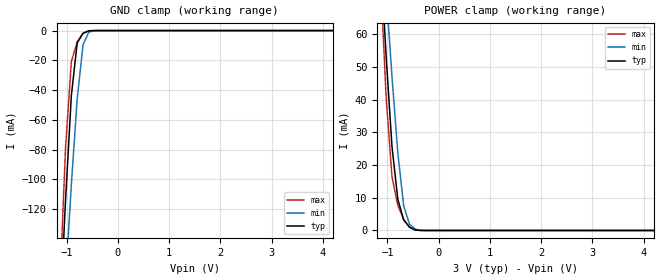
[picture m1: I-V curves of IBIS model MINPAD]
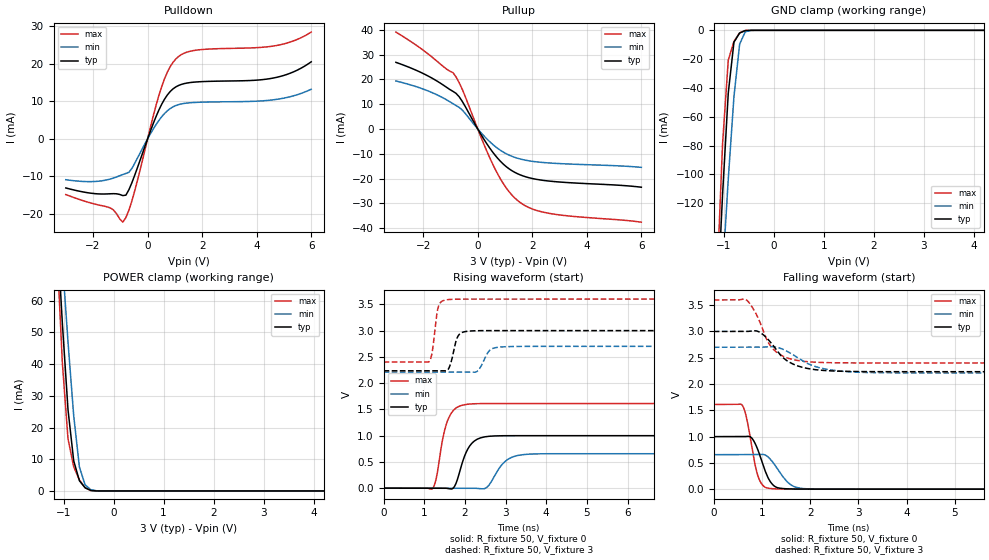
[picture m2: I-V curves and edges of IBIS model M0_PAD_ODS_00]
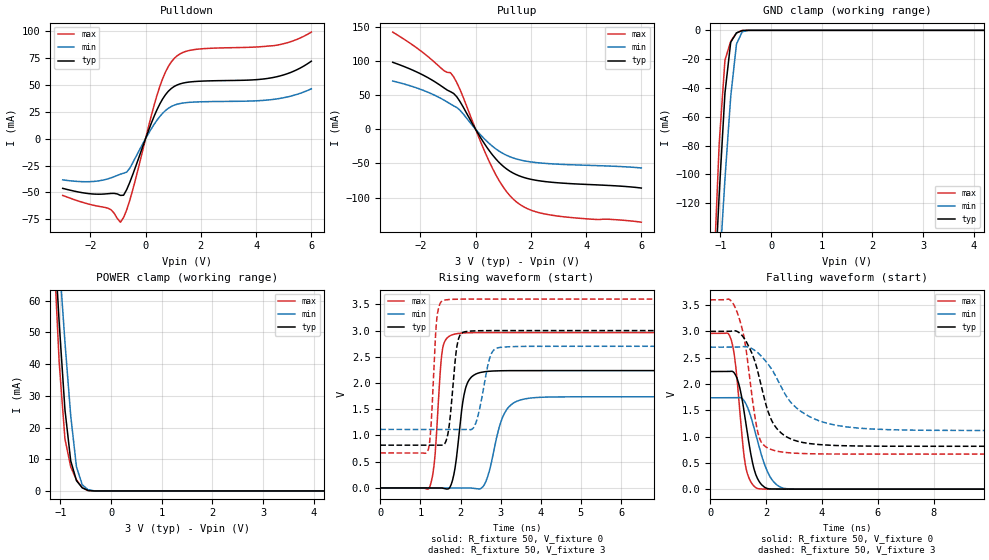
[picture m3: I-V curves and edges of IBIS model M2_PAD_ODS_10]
| Created by SiliconSmart  O-2018.09-SP2-3
[IBIS Ver]   4.0
[File Name]   as31b32bc_3p0_rev1p4.ibs
[File Rev]   1.4
[Date]   Thursday Mar 21 2024
|[Source]   Avalanche Team
|[Notes]   Generated IBIS models from Silicon Smart
|[Rev 1.0]  Initial Release based on extracted netlist
|   Characterization
|[Rev 1.1]  Recharacterization with Hspice, run in high accuracy mode
|[Rev 1.2]  Recharacterization with Hspice, run with parameters inline
|   with the datasheet
|[Rev 1.3]  Recharacterization with Hspice, run with updated VIH/VIL
|   in parallel with datasheet rev X.7
|[Rev 1.4]  Update the pin to the package pinout assignment
|[Disclaimer]   THE MODEL LIBRARIES ARE PROVIDED AS IS.
|[Copyright]   Copyright 2019, Avalanche Technology., All Rights Reserved
[Component]   AS301GB32_BGA
[Manufacturer] Avalanche Technology
| CONTENT :
| This file contains IBIS MODEL for PSRAM device
| AS301GB32
| USAGE :
| The models are derived for the 2.7V to 3.6V I/O Operation.
| Temperatures for model generation: typ: 25, max: -40, min: 125
| Voltages : typ: 3.0V, min: 2.7V, max: 3.6V
| PACKAGES SUPPORTED :
| 142-ball FBGA (15mm x 17mm)
| VERIFICATION
| Errors  : 0
| Warnings: 16
| All warnings due to non-monotonic data:
[Package]
R_pkg  0   0   0
L_pkg  0   0   0
C_pkg  0   0   0
[Pin]   signal_name   model_name   R_pin   L_pin   C_pin
P8   E#   MINPAD   0.254	7.307E-9	1.178E-12
P7   G#   MINPAD   0.243	7.052E-9	1.094E-12
J2   CR#   MINPAD   0.547	10.386E-9	1.789E-12
K3   PG#   MINPAD   0.451	10.329E-9	1.676E-12
M8   W#   MINPAD   0.377	9.020E-9	1.417E-12
M2   ADDR_26   MINPAD   0.425	9.037E-9	1.604E-12
L4   ADDR_25   MINPAD   0.419	9.644E-9	1.527E-12
K13   ADDR_24   MINPAD   0.495	9.978E-9	1.745E-12
M3   ADDR_23   MINPAD   0.371	9.313E-9	1.466E-12
L3   ADDR_22   MINPAD   0.412	9.753E-9	1.540E-12
M7   ADDR_21   MINPAD   0.368	8.765E-9	1.384E-12
P12   ADDR_20   MINPAD   0.287	8.287E-9	1.639E-12
L12   ADDR_19   MINPAD   0.424	10.320E-9	1.620E-12
N11   ADDR_18   MINPAD   0.338	8.691E-9	1.470E-12
N6   ADDR_17   MINPAD   0.309	8.196E-9	1.279E-12
P6   ADDR_16   MINPAD   0.256	7.462E-9	1.204E-12
L13   ADDR_15   MINPAD   0.463	10.719E-9	1.740E-12
M13   ADDR_14   MINPAD   0.421	10.290E-9	1.689E-12
P10   ADDR_13   MINPAD   0.262	7.671E-9	1.349E-12
N10   ADDR_12   MINPAD   0.340	8.540E-9	1.360E-12
M12   ADDR_11   MINPAD   0.402	9.876E-9	1.604E-12
N13   ADDR_10   MINPAD   0.399	9.819E-9	1.696E-12
L11   ADDR_9   MINPAD   0.443	9.732E-9	1.569E-12
M11   ADDR_8   MINPAD   0.436	9.682E-9	1.671E-12
P5   ADDR_7   MINPAD   0.253	7.464E-9	1.277E-12
P3   ADDR_6   MINPAD   0.279	8.031E-9	1.557E-12
N5   ADDR_5   MINPAD   0.313	8.320E-9	1.359E-12
N4   ADDR_4   MINPAD   0.329	8.138E-9	1.428E-12
M4   ADDR_3   MINPAD   0.379	8.543E-9	1.406E-12
N2   ADDR_2   MINPAD   0.378	9.572E-9	1.637E-12
N9   ADDR_1   MINPAD   0.315	8.416E-9	1.305E-12
M9   ADDR_0   MINPAD   0.403	9.225E-9	1.473E-12
E2   DQ_31   MIOPAD   0.365	8.798E-9	1.454E-12
F2   DQ_30   MIOPAD   0.418	9.057E-9	1.576E-12
D2   DQ_29   MIOPAD   0.358	8.697E-9	1.520E-12
E3   DQ_28   MIOPAD   0.348	8.812E-9	1.441E-12
E12   DQ_27   MIOPAD   0.327	8.506E-9	1.443E-12
D10   DQ_26   MIOPAD   0.309	7.715E-9	1.264E-12
C9   DQ_25   MIOPAD   0.279	7.395E-9	1.219E-12
C7   DQ_24   MIOPAD   0.252	6.802E-9	1.108E-12
G4   DQ_23   MIOPAD   0.455	10.071E-9	1.775E-12
G3   DQ_22   MIOPAD   0.457	10.100E-9	1.750E-12
F13   DQ_21   MIOPAD   0.377	9.387E-9	1.566E-12
D13   DQ_20   MIOPAD   0.295	8.231E-9	1.460E-12
C10   DQ_19   MIOPAD   0.293	7.553E-9	1.298E-12
E8   DQ_18   MIOPAD   0.393	8.323E-9	1.436E-12
F6   DQ_17   MIOPAD   0.425	8.913E-9	1.517E-12
E5   DQ_16   MIOPAD   0.379	8.982E-9	1.460E-12
E13   DQ_15   MIOPAD   0.363	8.555E-9	1.474E-12
G11   DQ_14   MIOPAD   0.475	9.536E-9	1.630E-12
E10   DQ_13   MIOPAD   0.404	8.563E-9	1.453E-12
F9   DQ_12   MIOPAD   0.409	9.347E-9	1.513E-12
C8   DQ_11   MIOPAD   0.257	6.782E-9	1.111E-12
C6   DQ_10   MIOPAD   0.238	7.000E-9	1.114E-12
D6   DQ_9   MIOPAD   0.292	7.776E-9	1.248E-12
D4   DQ_8   MIOPAD   0.305	7.782E-9	1.343E-12
G12   DQ_7   MIOPAD   0.502	10.055E-9	1.687E-12
C12   DQ_6   MIOPAD   0.275	7.857E-9	1.346E-12
D11   DQ_5   MIOPAD   0.286	7.835E-9	1.360E-12
D9   DQ_4   MIOPAD   0.306	8.035E-9	1.299E-12
E7   DQ_3   MIOPAD   0.384	8.178E-9	1.375E-12
C5   DQ_2   MIOPAD   0.231	6.786E-9	1.150E-12
D5   DQ_1   MIOPAD   0.307	7.698E-9	1.346E-12
C3   DQ_0   MIOPAD   0.267	7.420E-9	1.241E-12
G13   INT#   MIOPAD   0.480	10.704E-9	1.759E-12
F10   VSSIO   GND   NA   NA   NA
L10   VSSIO   GND   NA   NA   NA
E9   VSSIO   GND   NA   NA   NA
L9   VSSIO   GND   NA   NA   NA
F8   VSSIO   GND   NA   NA   NA
L8   VSSIO   GND   NA   NA   NA
F7   VSSIO   GND   NA   NA   NA
L7   VSSIO   GND   NA   NA   NA
E6   VSSIO   GND   NA   NA   NA
L6   VSSIO   GND   NA   NA   NA
G5   VSSIO   GND   NA   NA   NA
A14   VSS   GND   NA   NA   NA
B14   VSS   GND   NA   NA   NA
C14   VSS   GND   NA   NA   NA
H13   VSS   GND   NA   NA   NA
R14   VSS   GND   NA   NA   NA
T14   VSS   GND   NA   NA   NA
A13   VSS   GND   NA   NA   NA
T13   VSS   GND   NA   NA   NA
A12   VSS   GND   NA   NA   NA
G10   VSS   GND   NA   NA   NA
H10   VSS   GND   NA   NA   NA
J10   VSS   GND   NA   NA   NA
K10   VSS   GND   NA   NA   NA
F5   VSS   GND   NA   NA   NA
L5   VSS   GND   NA   NA   NA
A2   VSS   GND   NA   NA   NA
T2   VSS   GND   NA   NA   NA
A1   VSS   GND   NA   NA   NA
B1   VSS   GND   NA   NA   NA
R1   VSS   GND   NA   NA   NA
T1   VSS   GND   NA   NA   NA
F12   VCCIO   POWER   NA   NA   NA
J12   VCCIO   POWER   NA   NA   NA
E11   VCCIO   POWER   NA   NA   NA
M10   VCCIO   POWER   NA   NA   NA
D8   VCCIO   POWER   NA   NA   NA
N8   VCCIO   POWER   NA   NA   NA
D7   VCCIO   POWER   NA   NA   NA
N7   VCCIO   POWER   NA   NA   NA
M5   VCCIO   POWER   NA   NA   NA
E4   VCCIO   POWER   NA   NA   NA
F3   VCCIO   POWER   NA   NA   NA
J3   VCCIO   POWER   NA   NA   NA
C13   VCC   POWER   NA   NA   NA
P13   VCC   POWER   NA   NA   NA
D12   VCC   POWER   NA   NA   NA
N12   VCC   POWER   NA   NA   NA
C11   VCC   POWER   NA   NA   NA
F11   VCC   POWER   NA   NA   NA
H11   VCC   POWER   NA   NA   NA
J11   VCC   POWER   NA   NA   NA
K11   VCC   POWER   NA   NA   NA
P11   VCC   POWER   NA   NA   NA
C4   VCC   POWER   NA   NA   NA
F4   VCC   POWER   NA   NA   NA
H4   VCC   POWER   NA   NA   NA
J4   VCC   POWER   NA   NA   NA
K4   VCC   POWER   NA   NA   NA
P4   VCC   POWER   NA   NA   NA
D3   VCC   POWER   NA   NA   NA
N3   VCC   POWER   NA   NA   NA
C2   VCC   POWER   NA   NA   NA
P2   VCC   POWER   NA   NA   NA
| IOPAD
[Model Selector] MIOPAD
| Model Description
M0_PAD_ODS_00   ODS_00
M1_PAD_ODS_01   ODS_01
M2_PAD_ODS_10   ODS_10
M3_PAD_ODS_11   ODS_11
| Models and submodels in the file (5): MINPAD (Input), M0_PAD_ODS_00 (I/O), M2_PAD_ODS_10 (I/O), M1_PAD_ODS_01 (I/O), M3_PAD_ODS_11 (I/O)
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[Model] MINPAD
Model_type Input
Enable   Active-High
Vinl  =  0.8
Vinh  =  2.2
| Capacitance  typ   min   max
C_comp   1.532639e-12   1.418869e-12   1.647023e-12
| Variables   typ   min   max
[GND Clamp Reference]   0   0   0
[POWER Clamp Reference]   3   2.7   3.6
[Pulldown Reference]   0   0   0
[Pullup Reference]   3   2.7   3.6
[Temperature Range]   25   125   -40
[Voltage Range]   3   2.7   3.6
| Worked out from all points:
|   GND clamp passes 1 mA (typ) near -0.63 V on its own axis
|   POWER clamp passes 1 mA (typ) near -0.57 V on its own axis
[GND Clamp]
| Voltage   I(typ)   I(min)   I(max)
-3V       -1.712A    -1.49A     -2.05A
-1.138V   -196mA     -238.3mA   -175.4mA
-1.024V   -114.1mA   -169mA     -78.79mA
-910.3mV  -43.65mA   -103.4mA   -20.76mA
-796.6mV  -8.265mA   -46.07mA   -7.662mA
-682.8mV  -1.833mA   -9.55mA    -1.764mA
-569mV    -178.2uA   -969.7uA   -71.6uA
-455.2mV  -3.827uA   -72.47uA   -401.3nA
6V        0A         0A         0A
[POWER Clamp]
| Voltage   I(typ)   I(min)   I(max)
-3V       673.8mA    591mA      808.5mA
-1.138V   84.79mA    99.96mA    78.44mA
-1.024V   53.08mA    72.89mA    40.56mA
-910.3mV  25.62mA    46.98mA    16.4mA
-796.6mV  9.531mA    23.75mA    7.632mA
-682.8mV  3.235mA    7.564mA    3.468mA
-569mV    995.3uA    1.941mA    1.029mA
-455.2mV  154.7uA    390.4uA    112.5uA
-227.6mV  35.58nA    2.313uA    2.593nA
6V        0A         0A         0A
[Model] M0_PAD_ODS_00
Model_type I/O
Enable   Active-High
Vinl  =  0.8
Vinh  =  2.2
Vmeas =  1.5
Cref  =  30e-12
| Capacitance  typ   min   max
C_comp   1.536816e-12   1.424706e-12   1.652746e-12
| Variables   typ   min   max
[GND Clamp Reference]   0   0   0
[POWER Clamp Reference]   3   2.7   3.6
[Pulldown Reference]   0   0   0
[Pullup Reference]   3   2.7   3.6
[Temperature Range]   25   125   -40
[Voltage Range]   3   2.7   3.6
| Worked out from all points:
|   slope of the pulldown table from 0 to 0.45 V, typ, clamps not added: 54.7 ohm
|   slope of the pullup table from 0 to 0.45 V, typ, clamps not added: 57.3 ohm
|   GND clamp passes 1 mA (typ) near -0.63 V on its own axis
|   POWER clamp passes 1 mA (typ) near -0.57 V on its own axis
|   falling waveform, R_fixture 50, V_fixture 0: 20-80 % time 244ps typ, 320ps min, 198ps max; typ from 1 V to 0 V
|   falling waveform, R_fixture 50, V_fixture 3: 20-80 % time 499ps typ, 644ps min, 396ps max; typ from 3 V to 2.23 V
|   rising waveform, R_fixture 50, V_fixture 0: 20-80 % time 285ps typ, 362ps min, 248ps max; typ from 0 V to 1 V
|   rising waveform, R_fixture 50, V_fixture 3: 20-80 % time 146ps typ, 198ps min, 114ps max; typ from 2.23 V to 3 V
[GND Clamp]
| Voltage   I(typ)   I(min)   I(max)
-3V       -1.712A    -1.49A     -2.05A
-1.138V   -196mA     -238.3mA   -175.4mA
-1.024V   -114.1mA   -169mA     -78.8mA
-910.3mV  -43.65mA   -103.4mA   -20.77mA
-796.6mV  -8.267mA   -46.07mA   -7.668mA
-682.8mV  -1.833mA   -9.55mA    -1.767mA
-569mV    -178.4uA   -969.7uA   -71.94uA
-455.2mV  -3.831uA   -72.48uA   -403.8nA
6V        0A         0A         0A
[POWER Clamp]
| Voltage   I(typ)   I(min)   I(max)
-3V       673.8mA    591mA      808.5mA
-1.138V   84.79mA    99.96mA    78.44mA
-1.024V   53.08mA    72.89mA    40.56mA
-910.3mV  25.62mA    46.98mA    16.4mA
-796.6mV  9.531mA    23.75mA    7.632mA
-682.8mV  3.235mA    7.564mA    3.468mA
-569mV    995.3uA    1.941mA    1.029mA
-455.2mV  154.7uA    390.4uA    112.5uA
-227.6mV  35.58nA    2.313uA    2.593nA
6V        0A         0A         0A
[Pulldown]
| Voltage   I(typ)   I(min)   I(max)
-3V       -13.11mA   -10.91mA   -14.87mA
-1.366V   -14.66mA   -10.71mA   -18.44mA
-910.3mV  -15.13mA   -9.525mA   -22.23mA
-796.6mV  -15.02mA   -9.239mA   -20.99mA
-569mV    -11.56mA   -7.817mA   -16.37mA
206.9mV   4.069mA    2.602mA    6.097mA
517.2mV   9.226mA    5.888mA    13.93mA
724.1mV   11.7mA     7.479mA    17.77mA
1.034V    13.84mA    8.867mA    21.28mA
1.759V    15.14mA    9.703mA    23.62mA
4.614V    16.21mA    10.4mA     24.74mA
6V        20.54mA    13.21mA    28.45mA
[Pullup]
| Voltage   I(typ)   I(min)   I(max)
-3V       26.89mA    19.37mA    39.1mA
-1.821V   21.37mA    15.34mA    30.28mA
-910.3mV  15.2mA     10.23mA    22.74mA
-796.6mV  14.37mA    9.461mA    21.03mA
-569mV    11.16mA    7.659mA    16.04mA
206.9mV   -3.805mA   -2.558mA   -5.667mA
620.7mV   -10.37mA   -6.883mA   -15.82mA
1.034V    -15.12mA   -9.936mA   -23.64mA
1.552V    -18.5mA    -12.1mA    -29.65mA
2.069V    -20.15mA   -13.16mA   -32.55mA
2.69V     -21.11mA   -13.77mA   -34.19mA
6V        -23.51mA   -15.49mA   -37.63mA
[Ramp]
dV/dt_r   0.59988/0.284835n  0.393696/0.362182n  0.967082/0.24767n
dV/dt_f   0.45937/0.498633n  0.294233/0.644316n  0.719379/0.396117n
R_load = 50
[Falling Waveform]
R_fixture = 50
V_fixture = 0
V_fixture_min = 0
V_fixture_max = 0
| Time   V(typ)   V(min)   V(max)
0s        999.8mV    656.2mV    1.612V
592.6ps   1V         656.6mV    1.594V
662.7ps   1.002V     656.6mV    1.423V
775ps     985mV      656.7mV    887.5mV
920.8ps   732.5mV    658.3mV    236.4mV
1.05ns    387.5mV    655.1mV    44.33mV
1.221ns   87.43mV    516.2mV    8.708mV
1.592ns   4.378mV    87.01mV    1.102mV
2.018ns   780.3uV    4.7mV      706uV
21.88ns   13.06nV    -2.279uV   3.818uV
[Falling Waveform]
R_fixture = 50
V_fixture = 3
V_fixture_min = 2.7
V_fixture_max = 3.6
| Time   V(typ)   V(min)   V(max)
0s        3V         2.7V       3.6V
662.6ps   3.001V     2.701V     3.609V
930.9ps   2.997V     2.701V     3.233V
1.117ns   2.859V     2.709V     2.815V
1.233ns   2.732V     2.709V     2.664V
1.556ns   2.422V     2.604V     2.487V
2.006ns   2.286V     2.366V     2.42V
2.5ns     2.247V     2.259V     2.405V
3.502ns   2.235V     2.214V     2.401V
21.88ns   2.234V     2.21V      2.401V
[Rising Waveform]
R_fixture = 50
V_fixture = 0
V_fixture_min = 0
V_fixture_max = 0
| Time   V(typ)   V(min)   V(max)
0s        6.54nV     88.47nV    -73.19nV
1.207ns   -456.9uV   -520.5uV   -4.427mV
1.285ns   -486.5uV   -554.2uV   157.9mV
1.593ns   -8.932mV   -686.9uV   1.324V
1.775ns   80.53mV    -765.4uV   1.522V
2.069ns   743.7mV    -892.4uV   1.599V
2.519ns   980.4mV    5.17mV     1.611V
2.991ns   998.7mV    510.2mV    1.611V
3.605ns   998.9mV    648.6mV    1.611V
21.88ns   999.8mV    656.2mV    1.612V
[Rising Waveform]
R_fixture = 50
V_fixture = 3
V_fixture_min = 2.7
V_fixture_max = 3.6
| Time   V(typ)   V(min)   V(max)
0s        2.234V     2.21V      2.401V
1.115ns   2.235V     2.21V      2.406V
1.19ns    2.235V     2.21V      2.571V
1.354ns   2.235V     2.21V      3.473V
1.647ns   2.366V     2.21V      3.594V
1.836ns   2.903V     2.211V     3.599V
2.19ns    2.995V     2.21V      3.599V
2.637ns   2.999V     2.641V     3.599V
3.102ns   2.999V     2.696V     3.599V
21.88ns   3V         2.7V       3.6V
[Model] M2_PAD_ODS_10
Model_type I/O
Enable   Active-High
Vinl  =  0.8
Vinh  =  2.2
Vmeas =  1.5
Cref  =  30e-12
| Capacitance  typ   min   max
C_comp   1.536816e-12   1.424706e-12   1.652746e-12
| Variables   typ   min   max
[GND Clamp Reference]   0   0   0
[POWER Clamp Reference]   3   2.7   3.6
[Pulldown Reference]   0   0   0
[Pullup Reference]   3   2.7   3.6
[Temperature Range]   25   125   -40
[Voltage Range]   3   2.7   3.6
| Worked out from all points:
|   slope of the pulldown table from 0 to 0.45 V, typ, clamps not added: 15.7 ohm
|   slope of the pullup table from 0 to 0.45 V, typ, clamps not added: 15.7 ohm
|   GND clamp passes 1 mA (typ) near -0.63 V on its own axis
|   POWER clamp passes 1 mA (typ) near -0.57 V on its own axis
|   falling waveform, R_fixture 50, V_fixture 0: 20-80 % time 426ps typ, 590ps min, 315ps max; typ from 2.24 V to 0 V
|   falling waveform, R_fixture 50, V_fixture 3: 20-80 % time 746ps typ, 1.32ns min, 479ps max; typ from 3 V to 0.815 V
|   rising waveform, R_fixture 50, V_fixture 0: 20-80 % time 215ps typ, 348ps min, 149ps max; typ from 0 V to 2.24 V
|   rising waveform, R_fixture 50, V_fixture 3: 20-80 % time 158ps typ, 240ps min, 115ps max; typ from 0.815 V to 3 V
[GND Clamp]
| Voltage   I(typ)   I(min)   I(max)
-3V       -1.712A    -1.49A     -2.05A
-1.138V   -196mA     -238.3mA   -175.4mA
-1.024V   -114.1mA   -169mA     -78.8mA
-910.3mV  -43.65mA   -103.4mA   -20.77mA
-796.6mV  -8.267mA   -46.07mA   -7.668mA
-682.8mV  -1.833mA   -9.55mA    -1.767mA
-569mV    -178.4uA   -969.7uA   -71.94uA
-455.2mV  -3.831uA   -72.48uA   -403.8nA
6V        0A         0A         0A
[POWER Clamp]
| Voltage   I(typ)   I(min)   I(max)
-3V       673.8mA    591mA      808.5mA
-1.138V   84.79mA    99.96mA    78.44mA
-1.024V   53.08mA    72.89mA    40.56mA
-910.3mV  25.62mA    46.98mA    16.4mA
-796.6mV  9.531mA    23.75mA    7.632mA
-682.8mV  3.235mA    7.564mA    3.468mA
-569mV    995.3uA    1.941mA    1.029mA
-455.2mV  154.7uA    390.4uA    112.5uA
-227.6mV  35.58nA    2.313uA    2.593nA
6V        0A         0A         0A
[Pulldown]
| Voltage   I(typ)   I(min)   I(max)
-3V       -46.18mA   -38.31mA   -52.75mA
-1.366V   -51.15mA   -37.37mA   -64.58mA
-910.3mV  -52.72mA   -33.03mA   -77.58mA
-796.6mV  -52.54mA   -32.1mA    -73.2mA
-569mV    -40.41mA   -27.32mA   -57.03mA
206.9mV   14.21mA    9.09mA     21.22mA
517.2mV   32.23mA    20.57mA    48.54mA
724.1mV   40.88mA    26.13mA    61.99mA
1.034V    48.37mA    30.99mA    74.35mA
1.759V    52.94mA    33.91mA    82.6mA
4.614V    56.68mA    36.35mA    86.18mA
6V        71.86mA    46.21mA    98.85mA
[Pullup]
| Voltage   I(typ)   I(min)   I(max)
-3V       97.9mA     70.56mA    142mA
-1.821V   77.5mA     55.73mA    109.4mA
-910.3mV  54.96mA    36.99mA    82.75mA
-796.6mV  52.39mA    34.26mA    76.82mA
-569mV    40.81mA    28mA       58.57mA
103.4mV   -7.085mA   -4.779mA   -10.5mA
620.7mV   -37.92mA   -25.16mA   -57.78mA
1.034V    -55.27mA   -36.32mA   -86.42mA
1.552V    -67.66mA   -44.23mA   -108.4mA
2.069V    -73.7mA    -48.1mA    -119.1mA
2.793V    -77.6mA    -50.61mA   -125.8mA
6V        -85.91mA   -56.55mA   -135.8mA
[Ramp]
dV/dt_r   1.34189/0.214531n  1.04234/0.347547n  1.77705/0.14905n
dV/dt_f   1.31106/0.746016n  0.951015/1.316n  1.76015/0.479444n
R_load = 50
[Falling Waveform]
R_fixture = 50
V_fixture = 0
V_fixture_min = 0
V_fixture_max = 0
| Time   V(typ)   V(min)   V(max)
0s        2.236V     1.737V     2.962V
759.6ps   2.242V     1.738V     2.821V
866.2ps   2.205V     1.738V     2.533V
995.4ps   2.051V     1.741V     1.883V
1.254ns   1.331V     1.646V     471.7mV
1.53ns    464.2mV    1.239V     79.63mV
1.72ns    173.9mV    859.7mV    7.736mV
2.149ns   4.281mV    230.1mV    1.501mV
2.718ns   1.261mV    9.353mV    845.9uV
21.88ns   -788.6nV   325.5nV    -804nV
[Falling Waveform]
R_fixture = 50
V_fixture = 3
V_fixture_min = 2.7
V_fixture_max = 3.6
| Time   V(typ)   V(min)   V(max)
0s        3V         2.7V       3.6V
659.1ps   3.001V     2.7V       3.614V
907.4ps   3.01V      2.701V     3.438V
1.244ns   2.844V     2.711V     2.79V
1.71ns    2.222V     2.591V     1.067V
2.018ns   1.566V     2.415V     796.6mV
2.308ns   1.207V     2.186V     732.6mV
3.226ns   898.4mV    1.487V     679.2mV
4.9ns     824.5mV    1.183V     667.3mV
21.88ns   814.9mV    1.115V     666.4mV
[Rising Waveform]
R_fixture = 50
V_fixture = 0
V_fixture_min = 0
V_fixture_max = 0
| Time   V(typ)   V(min)   V(max)
0s        3.422nV    44.9nV     -42.68nV
1.217ns   809.2uV    -289.8uV   -4.263mV
1.357ns   902.5uV    -323.2uV   556.4mV
1.551ns   -3.954mV   -369.6uV   2.647V
1.916ns   686.9mV    -456.6uV   2.942V
2.257ns   2.103V     -1.49mV    2.959V
2.617ns   2.217V     98.55mV    2.961V
3.143ns   2.235V     1.484V     2.962V
3.73ns    2.236V     1.712V     2.962V
21.88ns   2.236V     1.737V     2.962V
[Rising Waveform]
R_fixture = 50
V_fixture = 3
V_fixture_min = 2.7
V_fixture_max = 3.6
| Time   V(typ)   V(min)   V(max)
0s        814.9mV    1.115V     666.4mV
1.189ns   814.4mV    1.116V     714.5mV
1.259ns   814.4mV    1.116V     1.121V
1.41ns    814.4mV    1.116V     3.235V
1.604ns   841.2mV    1.116V     3.581V
1.924ns   2.76V      1.116V     3.598V
2.159ns   2.983V     1.115V     3.599V
2.757ns   2.999V     2.539V     3.599V
3.026ns   2.999V     2.682V     3.599V
21.88ns   3V         2.7V       3.6V
